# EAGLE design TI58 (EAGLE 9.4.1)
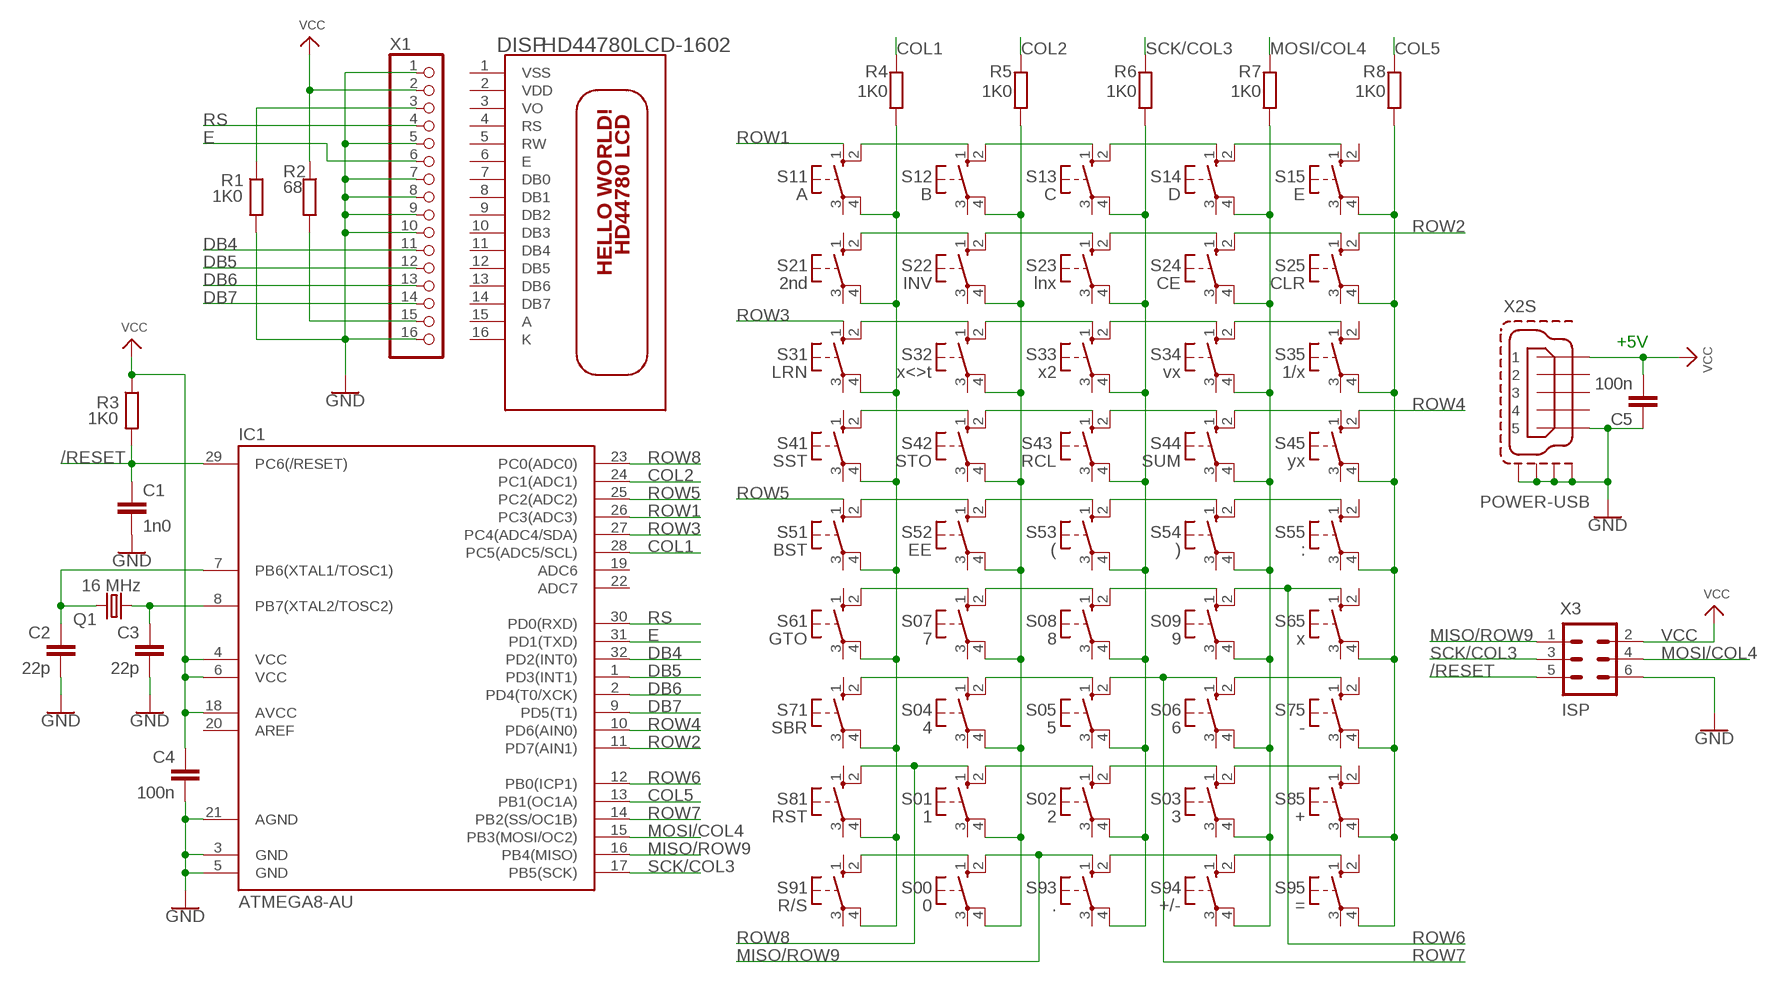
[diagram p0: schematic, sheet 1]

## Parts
C1  1n0  C-EU050-024X044  [C050-024X044]
C2  22p  C-EU050-024X044  [C050-024X044]
C3  22p  C-EU050-024X044  [C050-024X044]
C4  100n  C-EU050-024X044  [C050-024X044]
C5  100n  C-EU050-024X044  [C050-024X044]
DISP  HD44780LCD-1602  [LCD1602]
IC1  ATMEGA8-AU  [TQFP32-08]
Q1  16 MHz  CRYSTALHC49U-V  [HC49U-V]
R1  1K0  R-EU_0204/7  [0204/7]
R2  68  R-EU_0204/7  [0204/7]
R3  1K0  R-EU_0204/7  [0204/7]
R4  1K0  R-EU_0204/7  [0204/7]
R5  1K0  R-EU_0204/7  [0204/7]
R6  1K0  R-EU_0204/7  [0204/7]
R7  1K0  R-EU_0204/7  [0204/7]
R8  1K0  R-EU_0204/7  [0204/7]
S00  0  10-XX  [B3F-10XX]
S01  1  10-XX  [B3F-10XX]
S02  2  10-XX  [B3F-10XX]
S03  3  10-XX  [B3F-10XX]
S04  4  10-XX  [B3F-10XX]
S05  5  10-XX  [B3F-10XX]
S06  6  10-XX  [B3F-10XX]
S07  7  10-XX  [B3F-10XX]
S08  8  10-XX  [B3F-10XX]
S09  9  10-XX  [B3F-10XX]
S11  A  10-XX  [B3F-10XX]
S12  B  10-XX  [B3F-10XX]
S13  C  10-XX  [B3F-10XX]
S14  D  10-XX  [B3F-10XX]
S15  E  10-XX  [B3F-10XX]
S21  2nd  10-XX  [B3F-10XX]
S22  INV  10-XX  [B3F-10XX]
S23  lnx  10-XX  [B3F-10XX]
S24  CE  10-XX  [B3F-10XX]
S25  CLR  10-XX  [B3F-10XX]
S31  LRN  10-XX  [B3F-10XX]
S32  x<>t  10-XX  [B3F-10XX]
S33  x2  10-XX  [B3F-10XX]
S34  vx  10-XX  [B3F-10XX]
S35  1/x  10-XX  [B3F-10XX]
S41  SST  10-XX  [B3F-10XX]
S42  STO  10-XX  [B3F-10XX]
S43  RCL  10-XX  [B3F-10XX]
S44  SUM  10-XX  [B3F-10XX]
S45  yx  10-XX  [B3F-10XX]
S51  BST  10-XX  [B3F-10XX]
S52  EE  10-XX  [B3F-10XX]
S53  (  10-XX  [B3F-10XX]
S54  )  10-XX  [B3F-10XX]
S55  :  10-XX  [B3F-10XX]
S61  GTO  10-XX  [B3F-10XX]
S65  x  10-XX  [B3F-10XX]
S71  SBR  10-XX  [B3F-10XX]
S75  -  10-XX  [B3F-10XX]
S81  RST  10-XX  [B3F-10XX]
S85  +  10-XX  [B3F-10XX]
S91  R/S  10-XX  [B3F-10XX]
S93  .  10-XX  [B3F-10XX]
S94  +/-  10-XX  [B3F-10XX]
S95  =  10-XX  [B3F-10XX]
X1  PINHD-1X16/90  [1X16/90]
X2  POWER-USB  MINI-USB-SHIELD-UX60-MB-5ST  [UX60-MB-5ST]
X3  ISP  ML6  [ML6]

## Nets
/RESET: C1.1 IC1.29(PC6(/RESET)) R3.2 X3.5
COL1: IC1.28(PC5(ADC5/SCL)) R4.2
COL1B: R4.1 S11.4(P1) S21.4(P1) S31.4(P1) S41.4(P1) S51.4(P1) S61.4(P1) S71.4(P1) S81.4(P1) S91.4(P1)
COL2: IC1.24(PC1(ADC1)) R5.2
COL2B: R5.1 S00.4(P1) S01.4(P1) S04.4(P1) S07.4(P1) S12.4(P1) S22.4(P1) S32.4(P1) S42.4(P1) S52.4(P1)
COL3B: R6.1 S02.4(P1) S05.4(P1) S08.4(P1) S13.4(P1) S23.4(P1) S33.4(P1) S43.4(P1) S53.4(P1) S93.4(P1)
COL4B: R7.1 S03.4(P1) S06.4(P1) S09.4(P1) S14.4(P1) S24.4(P1) S34.4(P1) S44.4(P1) S54.4(P1) S94.4(P1)
COL5: IC1.13(PB1(OC1A)) R8.2
COL5B: R8.1 S15.4(P1) S25.4(P1) S35.4(P1) S45.4(P1) S55.4(P1) S65.4(P1) S75.4(P1) S85.4(P1) S95.4(P1)
DB4: IC1.32(PD2(INT0)) X1.11
DB5: IC1.1(PD3(INT1)) X1.12
DB6: IC1.2(PD4(T0/XCK)) X1.13
DB7: IC1.9(PD5(T1)) X1.14
E: IC1.31(PD1(TXD)) X1.6
GND: C1.2 C2.1 C3.1 C4.1 C5.1 IC1.3(GND) IC1.5(GND) IC1.21(AGND) R1.2 X1.1 X1.5 X1.7 X1.8 X1.9 X1.10 X1.16 X2.5 X2.M1(S:S1) X2.M2(S:S2) X2.M3(S:S3) X2.M4(S:S4) X3.6
LED: R2.2 X1.15
MISO/ROW9: IC1.16(PB4(MISO)) S00.2(S1) S93.1(S) X3.1
MOSI/COL4: IC1.15(PB3(MOSI/OC2)) R7.2 X3.4
N$1: S11.2(S1) S12.1(S)
N$2: S12.2(S1) S13.1(S)
N$3: S13.2(S1) S14.1(S)
N$4: S14.2(S1) S15.1(S)
N$5: S21.2(S1) S22.1(S)
N$6: S22.2(S1) S23.1(S)
N$7: S23.2(S1) S24.1(S)
N$8: S24.2(S1) S25.1(S)
N$9: S31.2(S1) S32.1(S)
N$10: S32.2(S1) S33.1(S)
N$11: S33.2(S1) S34.1(S)
N$12: S34.2(S1) S35.1(S)
N$13: S41.2(S1) S42.1(S)
N$14: S42.2(S1) S43.1(S)
N$15: S43.2(S1) S44.1(S)
N$16: S44.2(S1) S45.1(S)
N$17: S51.2(S1) S52.1(S)
N$18: S52.2(S1) S53.1(S)
N$19: S53.2(S1) S54.1(S)
N$21: S54.2(S1) S55.1(S)
N$22: S07.1(S) S61.2(S1)
N$23: S07.2(S1) S08.1(S)
N$24: S08.2(S1) S09.1(S)
N$26: S04.1(S) S71.2(S1)
N$27: S04.2(S1) S05.1(S)
N$29: S06.2(S1) S75.1(S)
N$31: S01.2(S1) S02.1(S)
N$32: S02.2(S1) S03.1(S)
N$33: S03.2(S1) S85.1(S)
N$34: S00.1(S) S91.2(S1)
N$36: S93.2(S1) S94.1(S)
N$37: S94.2(S1) S95.1(S)
N$43: C2.2 IC1.7(PB6(XTAL1/TOSC1)) Q1.2
N$44: C3.2 IC1.8(PB7(XTAL2/TOSC2)) Q1.1
ROW1: IC1.26(PC3(ADC3)) S11.1(S)
ROW2: IC1.11(PD7(AIN1)) S25.2(S1)
ROW3: IC1.27(PC4(ADC4/SDA)) S31.1(S)
ROW4: IC1.10(PD6(AIN0)) S45.2(S1)
ROW5: IC1.25(PC2(ADC2)) S51.1(S)
ROW6: IC1.12(PB0(ICP1)) S09.2(S1) S65.1(S)
ROW7: IC1.14(PB2(SS/OC1B)) S05.2(S1) S06.1(S)
ROW8: IC1.23(PC0(ADC0)) S01.1(S) S81.2(S1)
RS: IC1.30(PD0(RXD)) X1.4
SCK/COL3: IC1.17(PB5(SCK)) R6.2 X3.3
V0: R1.1 X1.3
VCC: C4.2 C5.2 IC1.4(VCC) IC1.6(VCC) IC1.18(AVCC) R2.1 R3.1 X1.2 X2.1 X3.2
Unconnected: DISP.1(VSS) DISP.2(VDD) DISP.3(VO) DISP.4(RS) DISP.5(RW) DISP.6(E) DISP.7(DB0) DISP.8(DB1) DISP.9(DB2) DISP.10(DB3) DISP.11(DB4) DISP.12(DB5) DISP.13(DB6) DISP.14(DB7) DISP.15(A) DISP.16(K) IC1.19(ADC6) IC1.20(AREF) IC1.22(ADC7) S00.3(P) S01.3(P) S02.3(P) S03.3(P) S04.3(P) S05.3(P) S06.3(P) S07.3(P) S08.3(P) S09.3(P) S11.3(P) S12.3(P) S13.3(P) S14.3(P) S15.2(S1) S15.3(P) S21.1(S) S21.3(P) S22.3(P) S23.3(P) S24.3(P) S25.3(P) S31.3(P) S32.3(P) S33.3(P) S34.3(P) S35.2(S1) S35.3(P) S41.1(S) S41.3(P) S42.3(P) S43.3(P) S44.3(P) S45.3(P) S51.3(P) S52.3(P) S53.3(P) S54.3(P) S55.2(S1) S55.3(P) S61.1(S) S61.3(P) S65.2(S1) S65.3(P) S71.1(S) S71.3(P) S75.2(S1) S75.3(P) S81.1(S) S81.3(P) S85.2(S1) S85.3(P) S91.1(S) S91.3(P) S93.3(P) S94.3(P) S95.2(S1) S95.3(P) X2.2 X2.3 X2.4

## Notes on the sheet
- +5V

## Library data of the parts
C1-C5 = rcl:C-EU: CAPACITOR, European symbol; SPICEPREFIX: C
DISP = adafruit:HD44780LCD: HD44780 LCD Standard character type LCDs, available in sizes from 8x1 to 40x4!
IC1 = atmega8:ATMEGA8
Q1 = crystal:CRYSTAL: CRYSTAL; OC_FARNELL: 1666969; OC_NEWARK: unknown
R1-R8 = rcl:R-EU_: RESISTOR, European symbol; SPICEPREFIX: R
S00 S01-S09 S11-S15 S21-S25 S31-S35 S41-S45 S51-S55 S61 S65 S71 S75 S81 S85 S91 S93-S95 = switch-omron2:10-XX: OMRON SWITCH; MPN: B3F-1000; OC_FARNELL: 176432; OC_NEWARK: 36M3542
X1 = pinhead:PINHD-1X16: PIN HEADER
X2 = con-hirose:MINI-USB-SHIELD-: MINI USB Connector Source: http://www.hirose.co.jp/cataloge_hp/e24000019.pdf; OC_FARNELL: unknown; OC_NEWARK: unknown
X3 = con-ml:ML6: HARTING; OC_FARNELL: unknown; OC_NEWARK: unknown

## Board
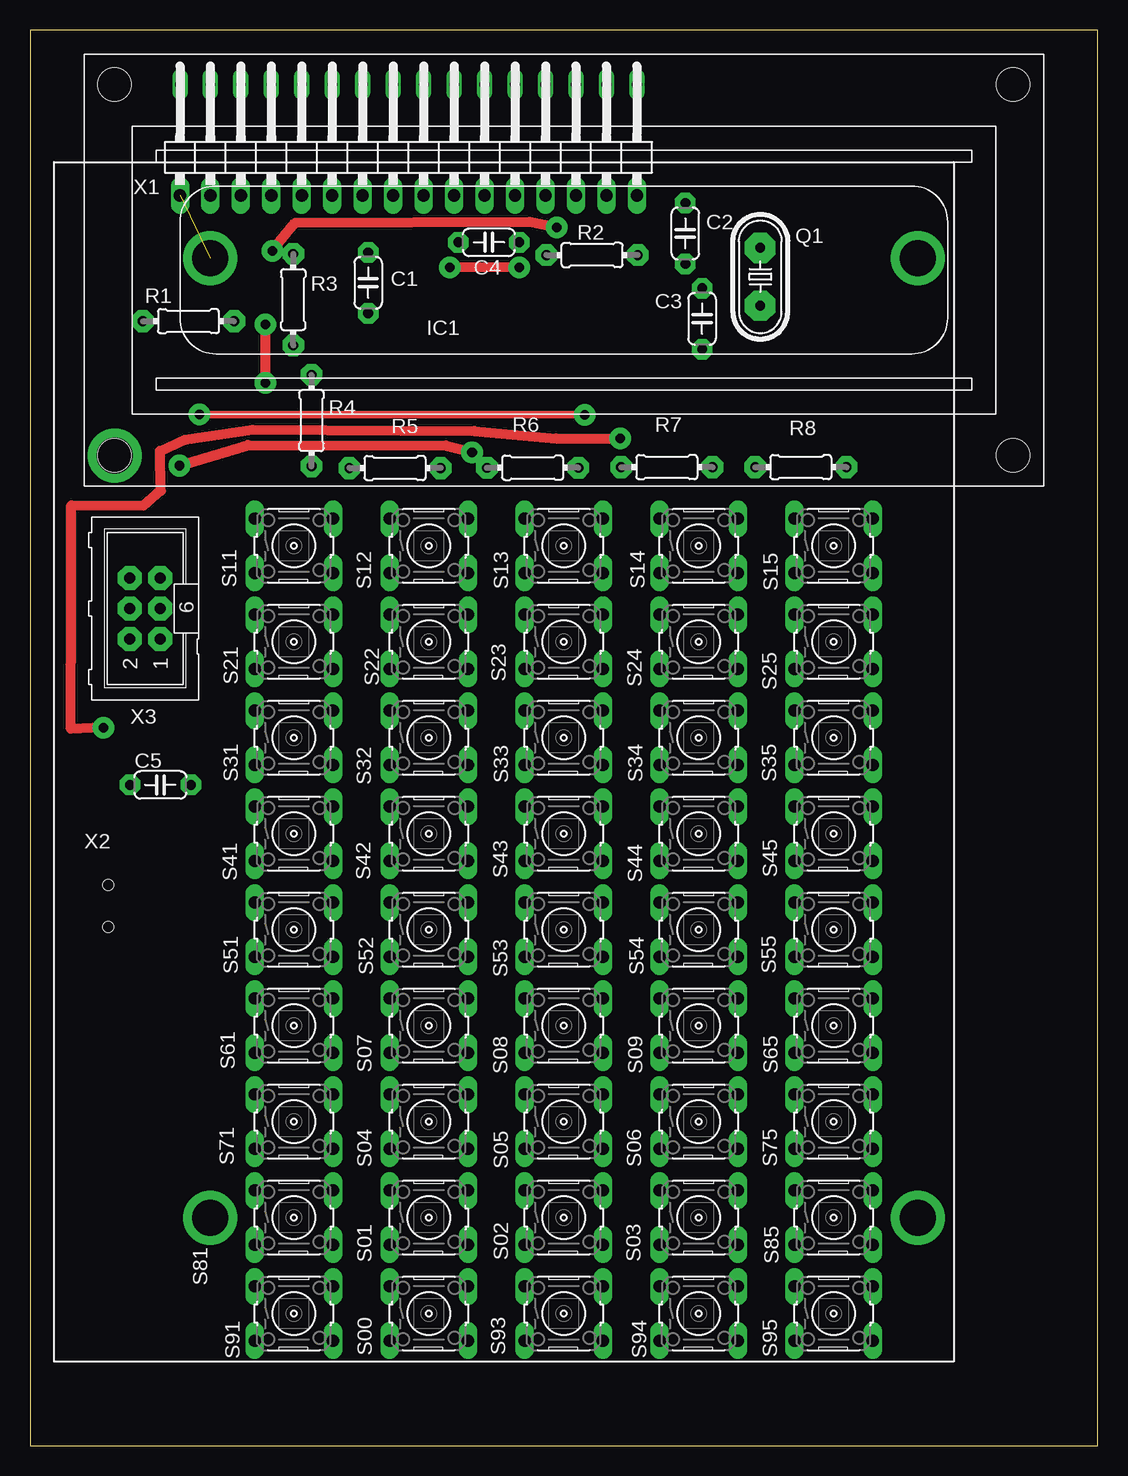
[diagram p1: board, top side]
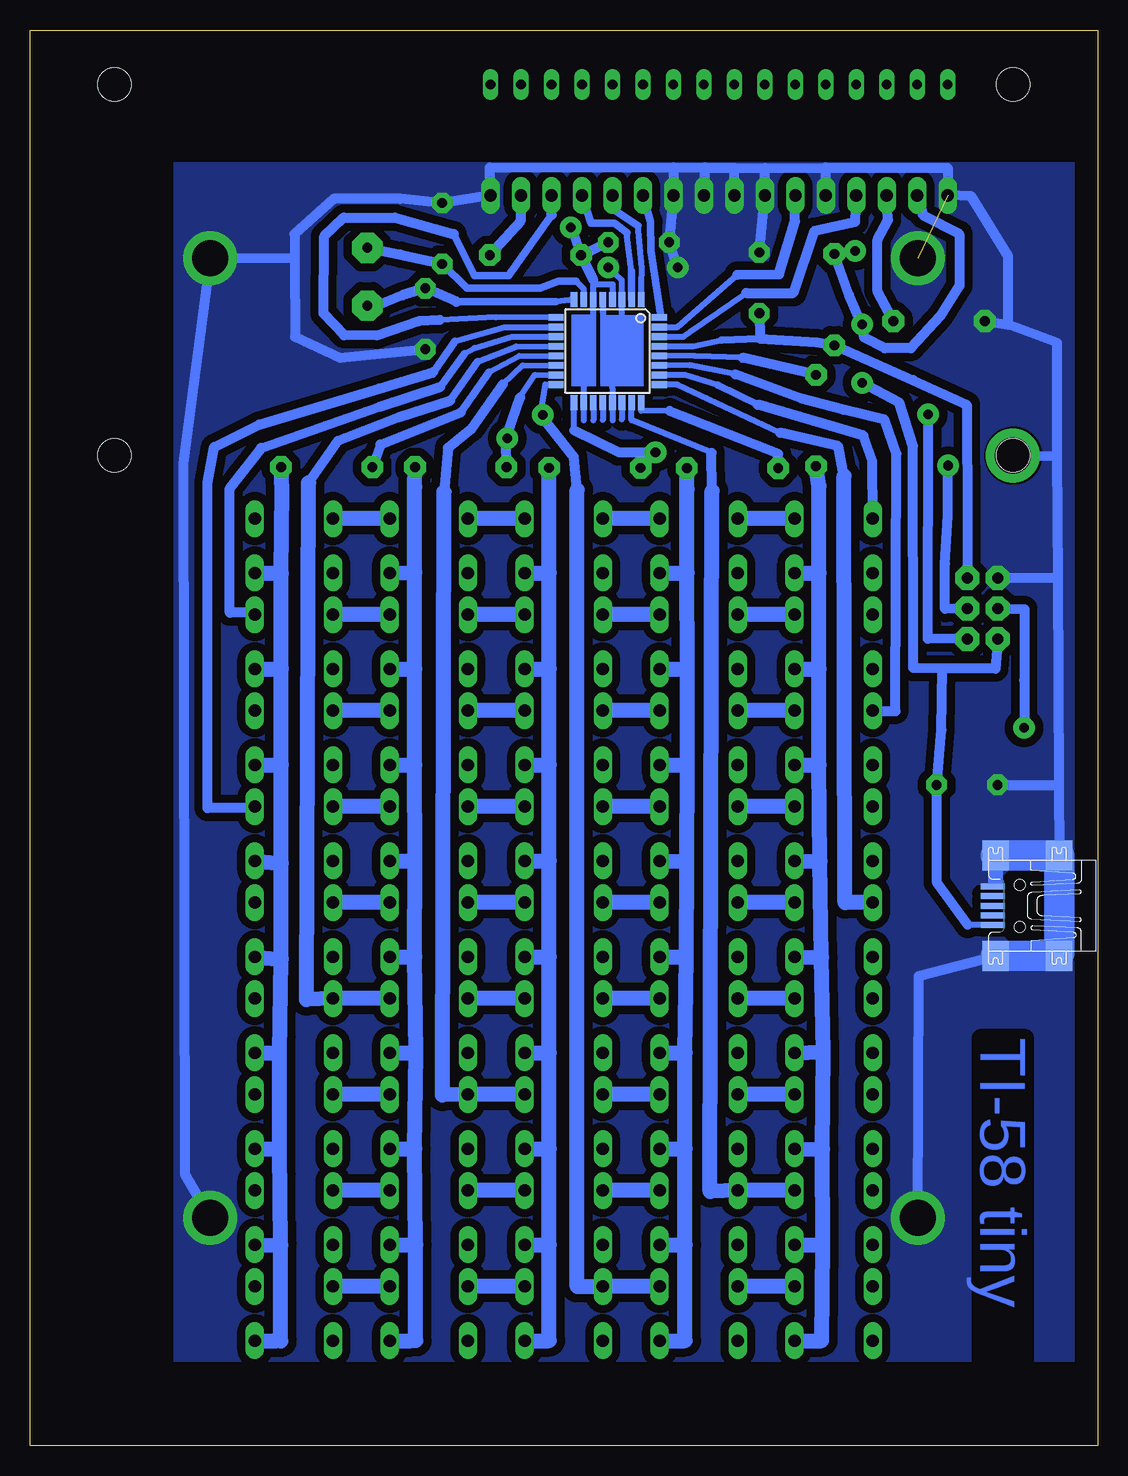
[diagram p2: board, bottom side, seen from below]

Size 89 x 118 mm. Coordinates in mm from the lower left corner, seen from the top.
Outline: 0,0 89,0 89,118 0,118 0,0
Copper layers (1*16): Top 0.035mm / dielectric 1.5mm / Bottom 0.035mm
Design rules "default": minimum track width 6mil, minimum drill 0.35mm, track to track 6mil, track to pad 6mil, pad to pad 6mil, via to via 6mil, smd to smd 6mil, copper to edge 40mil, drill to drill 6mil, minimum pad ring 10mil, minimum via ring 8mil, stop-mask expansion 4mil, vias tented up to drill 0mil, thermal gap 10mil

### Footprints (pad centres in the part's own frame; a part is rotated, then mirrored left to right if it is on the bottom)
C050-024X044 = drill 0.813 pad 1.7 octagon: 1 -2.54,0; 2 2.54,0
LCD1602 = drill 0.8 long: 1 8,33.46; 2 10.54,33.46; 3 13.08,33.46; 4 15.62,33.46; 5 18.16,33.46; 6 20.7,33.46; 7 23.24,33.46; 8 25.78,33.46; 9 28.32,33.46; 10 30.86,33.46; 11 33.4,33.46; 12 35.94,33.46; 13 38.48,33.46; 14 41.02,33.46; 15 43.56,33.46; 16 46.1,33.46 | hole 2.8: 2.54,2.54; 2.54,33.46; 77.46,33.46; 77.46,2.54
TQFP32-08 = smd 1.27 x 0.559: 1 -4.293,2.8; 2 -4.293,2; 3 -4.293,1.2; 4 -4.293,0.4; 5 -4.293,-0.4; 6 -4.293,-1.2; 7 -4.293,-2; 8 -4.293,-2.8; 17 4.293,-2.8; 18 4.293,-2; 19 4.293,-1.2; 20 4.293,-0.4; 21 4.293,0.4; 22 4.293,1.2; 23 4.293,2; 24 4.293,2.8 | smd 0.559 x 1.27: 9 -2.8,-4.293; 10 -2,-4.293; 11 -1.2,-4.293; 12 -0.4,-4.293; 13 0.4,-4.293; 14 1.2,-4.293; 15 2,-4.293; 16 2.8,-4.293; 25 2.8,4.293; 26 2,4.293; 27 1.2,4.293; 28 0.4,4.293; 29 -0.4,4.293; 30 -1.2,4.293; 31 -2,4.293; 32 -2.8,4.293
HC49U-V = drill 0.813 pad 2.54 octagon: 1 -2.413,0; 2 2.413,0
0204/7 = drill 0.813 pad 1.8 octagon: 1 -3.81,0; 2 3.81,0
B3F-10XX = drill 1.016 long: 1 -3.251,2.261; 2 3.251,2.261; 3 -3.251,-2.261; 4 3.251,-2.261
1X16/90 = drill 1.016 long: 1 -19.05,-3.81; 2 -16.51,-3.81; 3 -13.97,-3.81; 4 -11.43,-3.81; 5 -8.89,-3.81; 6 -6.35,-3.81; 7 -3.81,-3.81; 8 -1.27,-3.81; 9 1.27,-3.81; 10 3.81,-3.81; 11 6.35,-3.81; 12 8.89,-3.81; 13 11.43,-3.81; 14 13.97,-3.81; 15 16.51,-3.81; 16 19.05,-3.81
UX60-MB-5ST = smd 2 x 0.5: 1 2.25,1.6; 2 2.25,0.8; 3 2.25,0; 4 2.25,-0.8; 5 2.25,-1.6 | smd 2.2 x 2.5: M1 -3.3,-4.2; M2 -3.3,4.2; M3 2,4.2; M4 2,-4.2 | hole 0.9: 0,-1.75; 0,1.75
ML6 = drill 0.914 pad 2 octagon: 1 -2.54,-1.27; 2 -2.54,1.27; 3 0,-1.27; 4 0,1.27; 5 2.54,-1.27; 6 2.54,1.27

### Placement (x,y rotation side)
C1  28.19,96.93 90 top
C2  54.64,101.04 270 top
C3  56.03,93.93 90 top
C4  38.25,100.3 0 top
C5  10.87,55.07 0 top
DISP  4.5,80 0 top
IC1  40.84,91.24 270 bottom
Q1  60.88,97.43 90 top
R1  13.21,93.73 180 top
R2  46.86,99.24 0 top
R3  21.95,95.53 270 top
R4  23.47,85.45 90 top
R5  30.43,81.48 180 top
R6  41.91,81.51 180 top
R7  53.09,81.56 180 top
R8  64.26,81.56 180 top
S00  33.25,11 0 top
S01  33.25,19 0 top
S02  44.5,19 0 top
S03  55.75,19 0 top
S04  33.25,27 0 top
S05  44.5,27 0 top
S06  55.75,27 0 top
S07  33.25,35 0 top
S08  44.5,35 0 top
S09  55.75,35 0 top
S11  22,75 0 top
S12  33.25,75 0 top
S13  44.5,75 0 top
S14  55.75,75 0 top
S15  67,75 0 top
S21  22,67 0 top
S22  33.25,67 0 top
S23  44.5,67 0 top
S24  55.75,67 0 top
S25  67,67 0 top
S31  22,59 0 top
S32  33.25,59 0 top
S33  44.5,59 0 top
S34  55.75,59 0 top
S35  67,59 0 top
S41  22,51 0 top
S42  33.25,51 0 top
S43  44.5,51 0 top
S44  55.75,51 0 top
S45  67,51 0 top
S51  22,43 0 top
S52  33.25,43 0 top
S53  44.5,43 0 top
S54  55.75,43 0 top
S55  67,43 0 top
S61  22,35 0 top
S65  67,35 0 top
S71  22,27 0 top
S75  67,27 0 top
S81  22,19 0 top
S85  67,19 0 top
S91  22,11 0 top
S93  44.5,11 0 top
S94  55.75,11 0 top
S95  67,11 0 top
X1  31.55,108.03 0 top
X2  6.5,45 180 bottom
X3  9.6,69.77 90 top

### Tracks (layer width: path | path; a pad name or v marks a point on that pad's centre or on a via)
/RESET
  Bottom 0.508: IC1.29 33.71,91.64 31.34,92.13
  Bottom 0.61: 31.34,92.13 28.14,92.29
  Bottom 0.813: X3.5 10.85,76.76 10.9,86.77 15.39,88.82 R3.2 23.42,91.97 28.14,92.29 C1.1
COL1
  Bottom 0.508: 29.59,90.68 33.58,90.83 IC1.28
  Bottom 0.813: R4.2 29.59,90.68
COL1B
  Bottom 1.27: S91.4 22.99,8.74 22.91,16.74 | 22.91,16.74 22.94,24.69 | 22.94,24.69 22.86,32.82 | 22.86,32.82 23.01,40.69 | 23.01,40.69 23.14,48.69 | 23.14,48.69 23.22,56.74 | 23.22,56.74 23.22,64.74 | 23.22,64.74 23.22,72.74 | 23.22,72.74 23.22,80.01 R4.1 | S11.4 23.22,72.74 | S21.4 23.22,64.74 | S31.4 23.22,56.74 | S41.4 23.14,48.69 | S51.4 23.01,40.69 | S61.4 22.86,32.82 | S71.4 22.94,24.69 | S81.4 22.91,16.74
COL2
  Bottom 0.508: 35.69,86.23 38.05,86.26 IC1.24
  Bottom 0.813: R5.2 26.64,82.68 35.69,86.23
COL2B
  Bottom 1.27: S00.4 34.39,8.74 34.39,16.74 | 34.39,16.74 34.39,24.74 | 34.39,24.74 34.39,32.74 | 34.39,32.74 34.29,40.74 | 34.29,40.74 34.24,48.69 | 34.24,48.69 34.19,56.74 | 34.19,56.74 34.19,64.74 | 34.19,64.74 34.21,72.74 | 34.21,72.74 34.21,79.7 R5.1 | S12.4 34.21,72.74 | S22.4 34.19,64.74 | S32.4 34.19,56.74 | S42.4 34.24,48.69 | S52.4 34.29,40.74 | S07.4 34.39,32.74 | S04.4 34.39,24.74 | S01.4 34.39,16.74
COL3B
  Bottom 1.27: S93.4 45.72,8.74 45.72,16.74 | 45.72,16.74 45.72,24.74 | 45.72,24.74 45.72,32.74 | 45.72,32.74 45.72,40.74 | 45.72,40.74 45.72,48.74 | 45.72,48.74 45.72,56.74 | 45.72,56.74 45.72,64.74 | 45.72,64.74 45.72,72.74 | S13.4 45.72,72.74 | S23.4 45.72,64.74 | S33.4 45.72,56.74 | S43.4 45.72,48.74 | S53.4 45.72,40.74 | S08.4 45.72,32.74 | S05.4 45.72,24.74 | S02.4 45.72,16.74 | 45.72,72.74 R6.1
COL4B
  Bottom 0.813: 57.17,8.71 57.17,8.74 56.84,8.74
  Bottom 1.27: S94.4 57.17,8.74 | 56.84,8.74 56.84,16.74 | 56.84,16.74 56.92,24.74 | 56.92,24.74 56.82,32.74 | 56.82,32.74 56.92,40.74 | 56.92,40.74 56.9,48.74 | 56.9,48.74 56.92,56.74 | 56.92,56.74 56.92,64.74 | 56.92,64.74 56.92,72.79 | 56.92,72.79 56.92,79.91 R7.1 | S14.4 56.92,72.79 | S24.4 56.92,64.74 | S34.4 56.92,56.74 | S44.4 56.9,48.74 | S54.4 56.92,40.74 | S09.4 56.82,32.74 | S06.4 56.92,24.74 | S03.4 56.84,16.74
COL5
  Bottom 0.508: 50.72,89.48 48.21,90.83 IC1.13
  Bottom 0.61: 53.09,86.11 50.72,89.48
  Bottom 0.813: R8.2 59.79,83.44 53.09,86.11
COL5B
  Bottom 0.813: 68.4,8.74 68.1,8.69
  Bottom 1.27: S95.4 68.4,8.74 | 68.1,8.69 68.1,16.69 | 68.1,16.69 68.2,24.74 | 68.2,24.74 68.2,32.74 | 68.2,32.74 68.05,40.54 | 68.05,40.54 68.05,48.54 | 68.05,48.54 68.05,56.74 | 68.05,56.74 68.05,64.74 | 68.05,64.74 68.05,72.71 | 68.05,72.71 68,79.65 R8.1 | S85.4 68.1,16.69 | S75.4 68.2,24.74 | S65.4 68.2,32.74 | S55.4 68.05,40.54 | S45.4 68.05,48.54 | S35.4 68.05,56.74 | S25.4 68.05,64.74 | S15.4 68.05,72.71
DB4
  Bottom 0.508: IC1.32 36.45,94.36
  Bottom 0.61: 36.45,94.36 37.24,99.57 37.26,102.03 X1.11
DB5
  Bottom 0.508: IC1.1 38,98.12 38.3,101.68
  Bottom 0.61: 38.3,101.68 40.39,103.07
  Bottom 0.813: 40.39,103.07 X1.12
DB6
  Bottom 0.508: 38.86,97.89 39.22,100.81 39.24,101.09
  Bottom 0.61: IC1.2 38.86,97.89 | 39.24,101.09 40.26,101.88 42.22,101.88 X1.13
DB7
  Bottom 0.508: IC1.9 50.16,94.06 54.81,93.83
  Bottom 0.61: 53.67,100.99 51.94,97.51 49.1,97.51 45.52,102.56
  Bottom 0.813: 54.81,93.83 56.62,93.73 60.1,92.53 62.81,92.56 64.54,94.36 64.47,100.81 62.84,102.36 58.57,102.36 53.67,100.99 | 45.52,102.56 X1.14
E
  Bottom 0.508: IC1.31 35,93.24 30.02,97.59
  Bottom 0.813: 30.02,97.59 26.54,97.64 25.22,102.03 X1.6
GND  (via drill 0.8 pad 1.8, 3 pad 4.5)  (1 unrouted)
  Top 0.813: v40.79,98.22 v35,98.2
  Bottom 0.508: IC1.5 41.25,94.49 41.22,93.86 | 41.22,93.86 40.44,87.99 IC1.21 40.44,85.47 | 41.22,93.86 39.65,93.85 IC1.3 39.65,97.16 v40.79,98.22 | 8.51,47.02 X2.5
  Bottom 0.61: 3.2,41.02 X2.M2 3.79,40.8
  Bottom 0.813: 35.33,106.55 35.33,105.66 X1.10 C4.1 v35,98.2 | 35.33,106.55 32.69,106.53 | 32.69,106.53 30.25,106.51 | 30.25,106.51 27.71,106.49 | 27.71,106.49 22.66,106.53 | 22.66,106.53 12.5,106.5 X1.1 10.52,104.14 7.44,99.14 7.42,93.43 | X1.9 32.69,106.53 | X1.8 30.25,106.51 | 27.71,106.49 X1.7 C1.2 | X1.5 22.66,106.53 | 35.33,106.55 50.65,106.53 X1.16 C2.1 58.12,103.94 63.7,103.94 66.95,101.02 66.94,99.01 | 3.38,82.45 3.38,91.92 7.42,93.43 | R1.2 7.42,93.43 | 66.94,99.01 66.93,98.78 66.9,92.43 63.14,90.68 C3.1 | 66.94,99.01 v74,99 76.22,81.89 76.1,22.61 v74,19 | v15,19 14.91,39.14 X2.M3 | 3.38,82.45 v7.05,82.54 | 3.38,82.45 3.32,72.31 | 3.32,72.31 3.23,55.07 | 3.23,55.07 X2.M1 | 3.32,72.31 X3.6 | C5.1 3.23,55.07
  Bottom 1.27: X2.M4 8.51,47.02
  Bottom 2.54: 3.2,41.02 X2.M1 X2.M4 | X2.M3 3.79,40.8
  other vias: 15,99
  pour Bottom (isolate 0.7, no thermals): 2,7 77,7 77,107 2,107
LED
  Bottom 0.813: R2.2 48.08,102.11 X1.15
MISO/ROW9  (via drill 0.8 pad 1.8)
  Top 0.61: v14.12,85.95 19.51,85.93 v46.25,85.93
  Bottom 0.508: 46.15,85.58 46.33,86.67 46.02,88.44 IC1.16
  Bottom 0.61: v46.25,85.93 46.15,85.58
  Bottom 0.813: S93.1 41.25,13.23 | 43.38,79.68 43.66,82.4 46.15,85.58 | X3.1 14.16,67.25 v14.12,85.95
  Bottom 1.27: S00.2 S93.1 | 41.25,13.23 43.38,13.23 43.38,79.68
MOSI/COL4  (via drill 0.8 pad 1.8)
  Top 0.813: v6.12,59.84 3.4,59.74 3.43,70.69 3.45,78.38 9.5,78.36 10.9,79.6 10.85,82.91 12.9,83.84 18.57,84.68 37.03,84.58 43.89,83.95 v49.2,83.95
  Bottom 0.508: 48.13,87.38 46.89,89.26 IC1.15
  Bottom 0.61: 49.2,84.38 49.3,83.71 v49.2,83.95
  Bottom 0.813: R7.2 49.3,83.71 | 49.2,84.38 48.13,87.38 | X3.4 6.1,69.72 6.12,63.8 v6.12,59.84
N$1
  Bottom 1.27: S11.2 S12.1
N$2
  Bottom 1.27: S12.2 S13.1
N$3
  Bottom 1.27: S13.2 S14.1
N$4
  Bottom 1.27: S14.2 S15.1
N$5
  Bottom 1.27: S21.2 S22.1
N$6
  Bottom 1.27: S22.2 S23.1
N$7
  Bottom 1.27: S23.2 S24.1
N$8
  Bottom 1.27: S24.2 S25.1
N$9
  Bottom 1.27: S31.2 S32.1
N$10
  Bottom 1.27: S32.2 S33.1
N$11
  Bottom 1.27: S33.2 S34.1
N$12
  Bottom 1.27: S34.2 S35.1
N$13
  Bottom 1.27: S41.2 S42.1
N$14
  Bottom 1.27: S42.2 S43.1
N$15
  Bottom 1.27: S43.2 S44.1
N$16
  Bottom 1.27: S44.2 S45.1
N$17
  Bottom 1.27: S51.2 S52.1
N$18
  Bottom 1.27: S52.2 S53.1
N$19
  Bottom 1.27: S53.2 S54.1
N$20
  Bottom 0.508: 39.65,86.92 39.65,85.52
N$21
  Bottom 1.27: S54.2 S55.1
N$22
  Bottom 1.27: S61.2 S07.1
N$23
  Bottom 1.27: S07.2 S08.1
N$24
  Bottom 1.27: S08.2 S09.1
N$26
  Bottom 1.27: S71.2 S04.1
N$27
  Bottom 1.27: S04.2 S05.1
N$28
  Bottom 0.508: 41.25,86.79 41.25,85.5
N$29
  Bottom 1.27: S06.2 S75.1
N$30
  Bottom 0.508: 42.04,86.82 42.04,85.47
N$31
  Bottom 1.27: S01.2 S02.1
N$32
  Bottom 1.27: S02.2 S03.1
N$33
  Bottom 1.27: S03.2 S85.1
N$34
  Bottom 1.27: S91.2 S00.1
N$36
  Bottom 1.27: S93.2 S94.1
N$37
  Bottom 1.27: S94.2 S95.1
N$43
  Bottom 0.508: 43.46,97.05 42.85,96.42 IC1.7
  Bottom 0.61: C2.2 52.55,96.47 46.48,96.47 44.93,97.05 43.46,97.05
  Bottom 0.813: Q1.2 58.12,99.29 C2.2
N$44
  Bottom 0.508: IC1.8 45.14,95.35
  Bottom 0.61: 45.14,95.35 53.44,95.35
  Bottom 0.813: 53.44,95.35 C3.2 57.94,95.89 60.07,95.02 Q1.1
ROW1
  Bottom 0.508: 31.65,88.39 34.37,89.23 IC1.26
  Bottom 0.61: 28.32,86.77 31.65,88.39
  Bottom 0.813: S11.1 18.77,82.09 19.51,84.18 28.32,86.77
ROW2
  Bottom 0.508: 52.78,91.03 51.94,91.49 48.82,92.43 IC1.11
  Bottom 0.61: 54.79,88.27 52.78,91.03
  Bottom 0.813: S25.2 70.25,69.42 72.34,69.42 72.34,79.81 69.75,83.16 59.87,86.59 54.79,88.27
ROW3
  Bottom 0.508: 30.23,89.31 34.01,90.04 IC1.27
  Bottom 0.813: S31.1 18.75,61.21 16.84,61.21 16.76,82.65 17.78,85.52 21.18,86.33 24.69,87.27 30.23,89.31
ROW4
  Bottom 0.508: 53.54,92.05 49.45,93.22 IC1.10
  Bottom 0.61: 55.37,89.48 53.54,92.05
  Bottom 0.813: S45.2 70.25,53.14 74.19,53.14 74.19,80.26 73.64,83.24 69.88,85.11 59.89,88.11 55.37,89.48
ROW5
  Bottom 0.508: 26.47,84.43 35.03,88.44 IC1.25
  Bottom 0.813: 21.23,80.82 21.13,80.82 21.61,83.31 26.47,84.43
  Bottom 1.27: S51.1 21.06,45.26 21.13,80.82
ROW6
  Bottom 0.508: 51.69,90.35 48.46,91.62 IC1.12
  Bottom 0.61: 53.98,87.12 51.69,90.35
  Bottom 0.813: 65.56,80.26 65.79,80.26 63.32,83.77 58.27,85.72 53.98,87.12
  Bottom 1.27: S09.2 S65.1 65.94,37.18 65.79,80.26
ROW7
  Bottom 0.508: 49.58,88.47 47.9,90.04 IC1.14
  Bottom 0.813: 54.25,79.5 54.48,79.5 54.15,83.19 52.15,84.81 49.58,88.47
  Bottom 1.27: S05.2 S06.1 54.61,29.21 54.48,79.5
ROW8
  Bottom 0.508: 32.18,82.75 38.84,85.47 IC1.23
  Bottom 0.813: 32.08,79.6 32.13,79.6 32.18,82.75
  Bottom 1.27: S81.2 S01.1 32.31,21.18 32.13,79.6
RS
  Bottom 0.508: IC1.30 34.54,92.43 29.31,96.06
  Bottom 0.813: 29.31,96.06 25.38,96.06 23.6,101.27 20.19,102.01 X1.4
SCK/COL3  (via drill 0.8 pad 1.8)
  Top 0.813: v12.47,81.69 18.19,83.41 34.67,83.36 v36.85,82.8
  Bottom 0.508: 43.64,84.61 IC1.17
  Bottom 0.61: 38.02,81.84 38.09,82.79
  Bottom 0.813: R6.2 38.02,81.84 | 43.64,84.61 39.88,82.78 38.09,82.79 v36.85,82.8 | X3.3 12.72,69.75 12.72,73.48 12.5,77.5 v12.47,81.69
V0
  Bottom 0.813: R1.1 18.34,96.22 18.34,100.51 17.48,102.16 X1.3
VCC  (via drill 0.8 pad 1.8)
  Top 0.61: 19.63,93.83 v19.63,93.45
  Top 0.813: v19.63,88.59 19.63,93.83 | v20.19,99.59 22.12,101.93 41.68,102.01 v43.92,101.55
  Bottom 0.508: 42.04,96.77 IC1.6 42.04,93.78 42.82,88.14 IC1.18 42.85,85.47 | 42.04,96.77 40.44,96.77 IC1.4 | X2.1 10.82,43.41 | 42.04,96.77 42.04,97.18
  Bottom 0.813: X3.2 8.51,64.77 12.93,64.77 | X1.2 14.55,102.56 11.53,101.02 11.51,96.67 13.11,94.13 15.55,91.47 17.73,91.47 19.46,92.35 v19.63,93.45 20.73,95.94 R3.1 v20.19,99.59 | 12.93,64.77 15.37,64.82 15.39,83.34 16.54,86.94 v19.63,88.59 | v43.92,101.55 R2.1 | 10.82,43.41 13.39,46.93 13.41,52.45 C5.2 13.01,59.66 12.93,64.77 | 42.04,97.18 R2.1 | R2.1 C4.2
(copper drawn outside any net)
  shapes: Bottom area x2

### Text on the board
Bottom: TI-58 tiny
